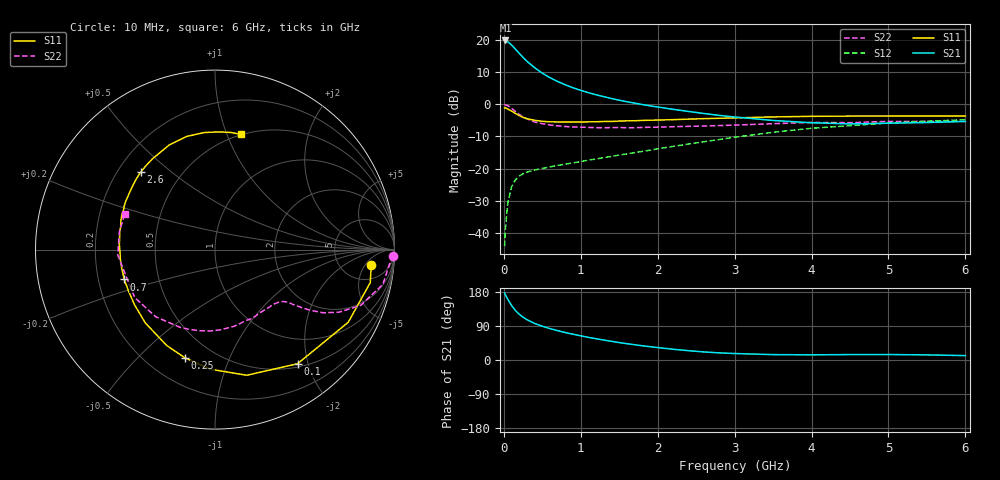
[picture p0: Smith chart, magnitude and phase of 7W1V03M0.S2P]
! Infineon Technologies  Discrete & RF Semiconductors
! BFS17W
! Si NPN RF Bipolar Junction Transistor in SOT323
! VCE = 1 V  IC = 3 mA
! Common Emitter S-Parameters:  August  1999
# GHz  S  MA  R  50
!  f  S11  S21  S12  S22
! GHz  MAG  ANG  MAG  ANG  MAG  ANG  MAG  ANG
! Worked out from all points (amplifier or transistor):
!   36 points, 10 MHz to 6 GHz, reference 50 ohm
!   highest |S21| = 19.9 dB at 20 MHz (marker M1)
!   |S21| within 3 dB of that: start of sweep to 161.8 MHz
!   unconditionally stable (mu >= 1): 640.6 MHz to end of sweep
!   at 250 MHz: K = 0.47, MSG = 18.1 dB, |S12| = -21.6 dB
!   at 1.4 GHz: K = 1.37, MAG = 5.4 dB, |S12| = -16.2 dB
!   at 6 GHz: K = 1.13, MAG = -2.4 dB, |S12| = -4.8 dB
!   S11 on the Smith chart (normalised r, x): 10 MHz: 10, -7; 100 MHz: 0.55, -1.83; 250 MHz: 0.35, -0.70; 700 MHz: 0.31, -0.14; 2.6 GHz: 0.29, +0.39; 6 GHz: 0.49, +1.12
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0.01  0.875 -5.7  9.799 176.7  0.0062 86.5  0.9948 -1.9
0.02  0.8844 -12.0  9.853 172.1  0.0114 87.1  0.9754 -4.8
0.05  0.8456 -28.6  9.411 160.5  0.0286 74.7  0.9552 -11.7
0.1  0.7849 -54.1  8.389 144.1  0.0517 62.3  0.8698 -20.9
0.15  0.7221 -75.8  7.228 130.7  0.0668 53.0  0.774 -26.8
0.2  0.6668 -92.3  6.218 120.7  0.0765 47.7  0.6975 -30.3
0.25  0.6256 -105.6  5.352 112.9  0.0828 43.2  0.635 -32.3
0.3  0.598 -116.8  4.678 106.5  0.0882 41.3  0.5926 -33.5
0.4  0.5636 -133.5  3.709 96.6  0.0949 38.8  0.5311 -35.1
0.5  0.5438 -145.5  3.054 89.1  0.1007 38.7  0.4987 -35.9
0.6  0.5341 -154.7  2.592 82.8  0.1062 39.4  0.4762 -37.4
0.7  0.5322 -161.8  2.264 77.4  0.1118 40.5  0.4617 -39.3
0.9  0.5301 -173.7  1.807 68.0  0.1226 42.9  0.4436 -43.8
1.1  0.5336 177.1  1.516 59.7  0.1351 45.2  0.437 -49.3
1.3  0.5403 169.2  1.313 52.5  0.1482 47.4  0.4316 -55.7
1.6  0.5535 159.8  1.095 43.0  0.1692 50.2  0.4317 -65.3
2.2  0.5771 143.8  0.836 28.4  0.2212 53.6  0.4484 -86.2
2.6  0.5983 133.9  0.72 21.3  0.2614 53.6  0.4597 -100.4
3.5  0.6365 113.6  0.56 14.2  0.3675 48.7  0.4994 -131.5
4.5  0.6549 95.3  0.495 14.3  0.4652 37.5  0.5183 -164.5
5.5  0.6587 82.3  0.52 13.5  0.5441 26.6  0.5417 169.7
6  0.6581 77.4  0.542 11.6  0.5764 21.3  0.5414 158.4
